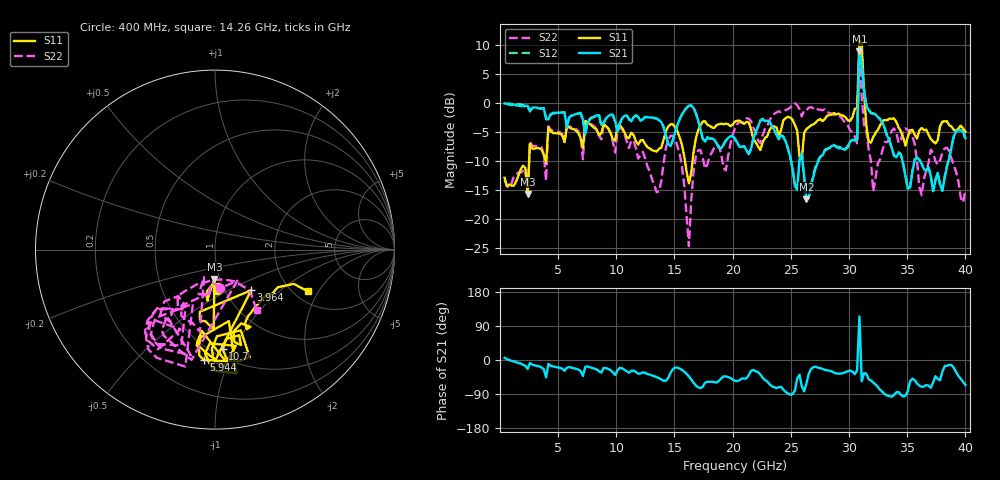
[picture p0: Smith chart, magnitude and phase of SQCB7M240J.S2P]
! Network Analyzer HP8722ES.07.66: Jul 25, 2000 Serial No. US39175408
! 27 Oct 2004  08:45:13
! Frequency  S11  S21  S12  S22
# HZ  S  DB R  50
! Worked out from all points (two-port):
!   201 points, 400 MHz to 40 GHz, reference 50 ohm
!   highest |S21| = 8.86 dB at 30.89 GHz (marker M1); lowest = -16.6 dB at 26.34 GHz (marker M2)
!   |S21| within 3 dB of the highest: 30.85 GHz to 31.11 GHz (261.1 MHz wide, 0.843 % of centre)
!   lowest |S11| = -15.7 dB at 2.38 GHz (marker M3), VSWR 1.39, Z = 47.1 - j15.8 ohm
!   |S11| at or under -10 dB: start of sweep to 2.511 GHz; 3.913 GHz to 3.976 GHz (62.35 MHz wide, 1.58 % of centre); 15.9 GHz to 16.55 GHz (654.7 MHz wide, 4.04 % of centre)
!   |S22| runs from -24.7 to 9.6 dB; largest |S21 - S12| = 0.91
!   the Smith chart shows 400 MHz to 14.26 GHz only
!   S11 on the Smith chart (normalised r, x): 400 MHz: 0.92, -0.44; 3.964 GHz: 1.32, -0.66; 5.944 GHz: 0.41, -0.81; 10.7 GHz: 0.56, -0.91; 14.26 GHz: 2.36, -1.61
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4e8  -12.92 -87.3  -0.12 5.6  -0.05 7.0  -13.25 -83.1
2.38e9  -15.72 -91.1  -0.51 -23.7  -0.65 -23.3  -15.64 -111.6
3.964e9  -10.36 -48.3  -2.69 -46.0  -2.87 -46.5  -13.42 -54.4
5.944e9  -4.19 -95.8  -2.52 -18.5  -2.57 -18.7  -4.06 -118.4
7.132e9  -7.84 -79.0  -2.89 -42.3  -3.03 -43.9  -9.72 -112.2
1.0696e10  -5.08 -85.5  -2.26 -25.6  -2.27 -25.6  -5.36 -132.9
1.3666e10  -7.93 -37.7  -3.03 -47.9  -2.99 -48.0  -15.25 -74.3
1.426e10  -4.95 -24.2  -5.67 -54.7  -5.68 -55.8  -7.79 -55.4
1.624e10  -13.88 -17.0  -0.55 -43.5  -0.51 -43.8  -24.68 108.7
1.7032e10  -4.80 19.1  -3.04 -72.1  -3.08 -72.6  -8.19 -14.4
2.02e10  -3.22 10.9  -6.20 -55.2  -6.26 -55.3  -4.39 3.0
2.4754e10  -2.43 -12.7  -7.85 -88.5  -8.03 -88.9  -1.09 -9.2
2.6338e10  -4.51 -107.1  -16.64 -62.2  -16.58 -63.6  -1.31 -16.2
2.6932e10  -3.73 -155.1  -12.71 -19.0  -12.35 -19.4  -0.93 -24.7
3.0694e10  -0.93 82.3  -6.49 -26.7  -6.26 -27.0  -6.98 -68.5
3.0892e10  10.64 -29.5  8.86 114.8  10.71 103.1  9.57 -55.9
3.109e10  10.25 -6.0  6.39 -56.0  6.29 -55.6  0.97 -146.3
3.1288e10  2.02 -26.9  2.16 -34.5  2.18 -34.4  -3.79 -83.8
3.1486e10  -3.93 -21.0  -0.46 -36.4  -0.34 -36.8  -4.77 -57.7
3.208e10  -5.92 -34.4  -1.89 -59.4  -1.83 -59.4  -15.26 -45.3
3.3466e10  -2.73 -90.1  -6.44 -95.2  -6.61 -94.0  -6.38 8.1
4e10  -4.99 -107.2  -6.11 -65.6  -6.12 -64.4  -15.10 -56.5
